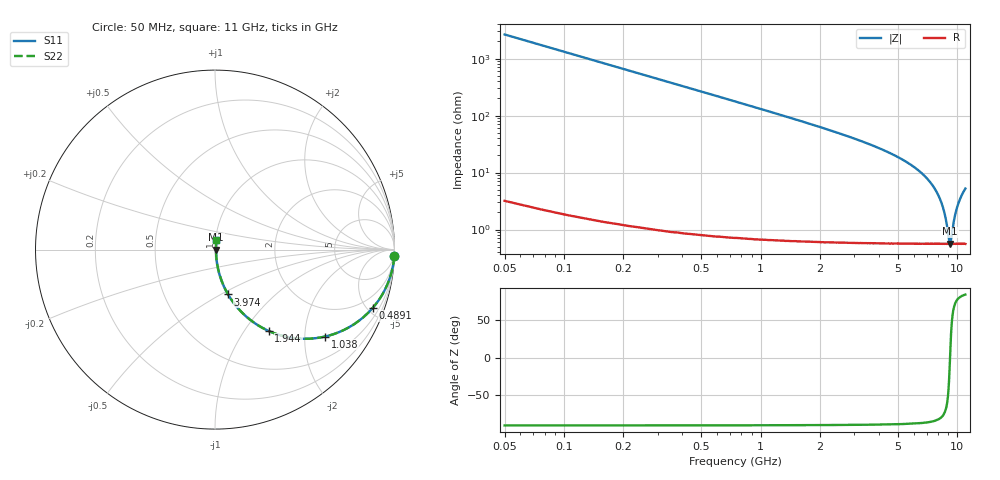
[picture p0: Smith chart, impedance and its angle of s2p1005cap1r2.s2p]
!	AVX	Thin	Film	Operation
!	Date:	March 2012
!	Description: Ultra-Miniature 01005 Size ACCU - P® Thin Film RF / Microwave Capacitor
!	Part Number:  C005YK1R2ABSTR
!	Serial	Measurements
#	MHz	S	db	R	50
!	S11	S21	S12	S22
!	dB	Phase	dB	Phase	dB	Phase	dB	Phase
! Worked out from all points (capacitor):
!   400 points, 50 MHz to 11 GHz, reference 50 ohm
!   read as one part in series: C = 1.2 pF near 104.9 MHz
!   lowest |Z| = 564 mohm at 9.189 GHz (marker M1)
!   series resonance near 9.189 GHz, so ESL is about 250 pH
!   S11 on the Smith chart (normalised r, x): 50 MHz: 1, -53; 489.1 MHz: 1.02, -5.41; 1.038 GHz: 1.01, -2.52; 1.944 GHz: 1.01, -1.30; 3.974 GHz: 1.01, -0.54; 11 GHz: 1.01, +0.10
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50  -0.01 -2.2  -28.48 87.8  -28.48 87.8  -0.01 -2.2
104.887  -0.03 -4.5  -22.07 85.4  -22.07 85.4  -0.03 -4.5
187.218  -0.09 -8.0  -17.09 81.9  -17.09 81.9  -0.09 -8.0
324.436  -0.26 -13.8  -12.48 76.1  -12.48 76.1  -0.26 -13.8
489.098  -0.56 -20.3  -9.21 69.6  -9.21 69.6  -0.56 -20.3
1037.97  -2.14 -38.3  -4.16 51.4  -4.16 51.4  -2.14 -38.3
1888.722  -5.10 -55.7  -1.66 33.8  -1.66 33.8  -5.10 -55.7
1943.609  -5.29 -56.5  -1.57 32.9  -1.57 32.9  -5.29 -56.5
2684.586  -7.75 -65.1  -0.85 24.2  -0.85 24.2  -7.75 -65.1
3700  -10.87 -72.3  -0.42 16.6  -0.42 16.6  -10.87 -72.3
3974.436  -11.69 -73.7  -0.35 15.1  -0.35 15.1  -11.69 -73.7
5538.722  -16.48 -79.3  -0.15 8.6  -0.15 8.6  -16.48 -79.3
7350  -23.78 -81.3  -0.07 3.7  -0.07 3.7  -23.78 -81.3
7981.203  -27.76 -79.8  -0.06 2.3  -0.06 2.3  -27.76 -79.8
8447.744  -32.11 -75.6  -0.05 1.4  -0.05 1.4  -32.11 -75.6
8749.624  -36.40 -67.5  -0.05 0.8  -0.05 0.8  -36.40 -67.5
9106.391  -44.20 -24.7  -0.05 0.1  -0.05 0.1  -44.20 -24.7
9188.722  -45.04 -0.0  -0.05 0.0  -0.05 0.0  -45.04 -0.0
9627.82  -36.76 66.6  -0.05 -0.8  -0.05 -0.8  -36.76 66.6
9929.699  -32.78 74.6  -0.05 -1.3  -0.05 -1.3  -32.78 74.6
10396.24  -28.89 79.0  -0.05 -2.0  -0.05 -2.0  -28.89 79.0
11000  -25.65 80.9  -0.06 -3.0  -0.06 -3.0  -25.65 80.9
